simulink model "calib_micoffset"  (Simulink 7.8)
settings: Solver=FixedStepDiscrete  SolverMode=SingleTasking  StartTime=0.0  StopTime=inf  FixedStep=Ts  RelTol=1e-3
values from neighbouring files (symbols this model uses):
  amp_gain_factor = 0.73316    [hybrid_wind.m]    (also in measurements.m = 0.73312)
  Ampl_chirp = maxoutputvoltage/4    (= 1.25)    [measurements.m]
  Ampl_chirp_F = maxLSvolts*Bl/Re    [measurements.m]
  Ampl_chirp_U = maxoutputvoltage *amp_gain_factor*Bl/Re/(2*pi*fstop)*Sd/Mms    [measurements.m]
  HLL_d = c2d(HLL_c,Ts)    [hybrid_wind.m]    (also in measurements.m)
  maxoutputvoltage = 5    [hybrid_wind.m]    (also in measurements.m)
  sweep_time = runtime    (= 20)    [measurements.m]
  Ts = 25e-6    (= 2.5e-05)    [hybrid_wind.m]    (also in measurements.m)
undefined symbols (not defined in the file or in its folder): Bl, cell2mat, Mms, Re, Sd
libraries: dspsrcs4 x2, simulink x1

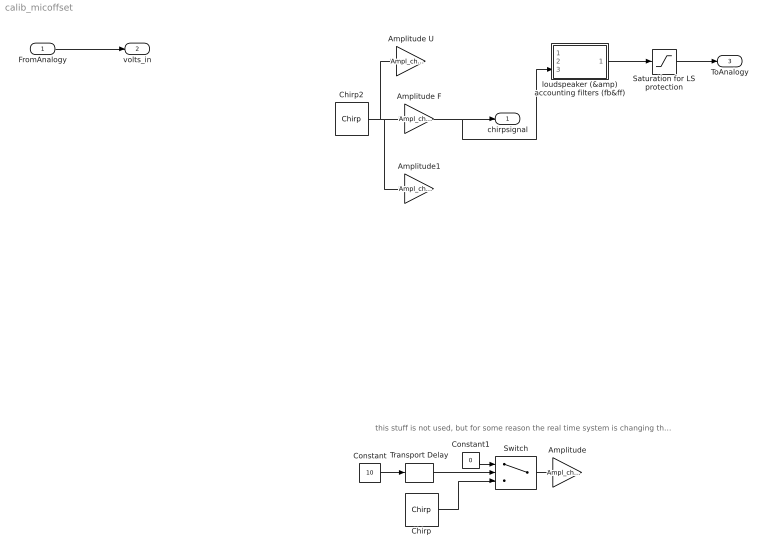
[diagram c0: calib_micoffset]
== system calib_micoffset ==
  note: this stuff is not used, but for some reason the real time system is changing the execution timing when the simulink patch is not complex enough!!
  FromAnalogy : Inport
  Amplitude : Gain  Gain=Ampl_chirp
  Amplitude F : Gain  Gain=Ampl_chirp_F
  Amplitude U : Gain  Gain=Ampl_chirp_U
  Amplitude1 : Gain  Gain=Ampl_chirp
  Chirp : dspsrcs4/Chirp  sweep=Linear  mode=Unidirectional  f0=fstart  f1=fstop  t1=sweep_time  Tsweep=sweep_time  phase=pi/2  Ts=Ts  spf=1  datatype=Single
  Chirp2 : dspsrcs4/Chirp  sweep=Linear  mode=Unidirectional  f0=fstart  f1=fstop  t1=sweep_time  Tsweep=sweep_time  phase=pi/2  Ts=Ts  spf=1  datatype=Double
  Constant : Constant  Value=10
  Constant1 : Constant  Value=0
  Saturation for LS protection : Saturate  UpperLimit=maxoutputvoltage  LowerLimit=-maxoutputvoltage
  Switch : Switch  Threshold=1
  Transport Delay : TransportDelay  DelayTime=sweep_time  BufferSize=8
  loudspeaker (&amp) accounting filters (fb&ff) : Subsystem
  chirpsignal : Outport
  volts_in : Outport  Port=2
  ToAnalogy : Outport  Port=3
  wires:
  FromAnalogy/1 -> volts_in/1
  Constant/1 -> Transport Delay/1
  Transport Delay/1 -> Switch/2
  Constant1/1 -> Switch/1
  Switch/1 -> Amplitude/1
  Chirp/1 -> Switch/3
  Amplitude/1 -> ?
  Chirp2/1 -> Amplitude F/1, Amplitude1/1, Amplitude U/1
  Saturation for LS protection/1 -> ToAnalogy/1
  loudspeaker (&amp) accounting filters (fb&ff)/1(V_amp_in) -> Saturation for LS protection/1
  Amplitude F/1 -> loudspeaker (&amp) accounting filters (fb&ff)/3(FLS), chirpsignal/1

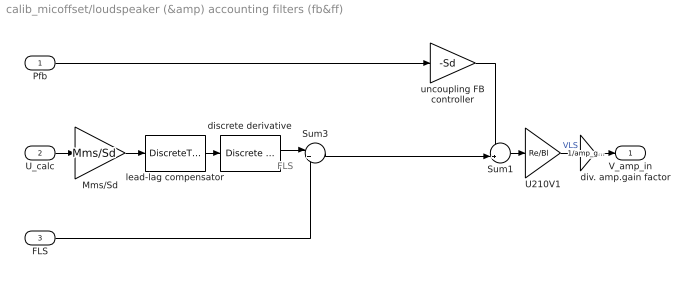
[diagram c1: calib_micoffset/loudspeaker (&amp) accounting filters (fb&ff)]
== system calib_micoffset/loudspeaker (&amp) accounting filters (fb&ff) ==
  note: FLS
  Pfb : Inport
  U_calc : Inport  Port=2
  FLS : Inport  Port=3
  Mms/Sd : Gain  Gain=Mms/Sd
  Sum1 : Sum  Inputs=-+|
  Sum3 : Sum  Inputs=|++
  U210V1 : Gain  Gain=Re/Bl
  discrete derivative : simulink/Discrete/Discrete Derivative  gainval=1.0  ICPrevScaledInput=0.0  InputProcessing=Inherited  OutMin=[]  OutMax=[]  OutDataType=fixdt(1, 16)  OutScaling=2^-10  DoSatur=off
  div. amp.gain factor : Gain  Gain=1/amp_gain_factor
  lead-lag compensator : DiscreteTransferFcn  Numerator=cell2mat(HLL_d.num)  Denominator=cell2mat(HLL_d.den)  SampleTime=Ts
  uncoupling FB controller : Gain  Gain=-Sd
  V_amp_in : Outport
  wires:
  Sum1/1 -> U210V1/1
  U210V1/1 -> div. amp.gain factor/1  "VLS"
  U_calc/1 -> Mms/Sd/1
  Pfb/1 -> uncoupling FB controller/1
  Mms/Sd/1 -> lead-lag compensator/1
  lead-lag compensator/1 -> discrete derivative/1
  div. amp.gain factor/1 -> V_amp_in/1
  Sum3/1 -> Sum1/2
  FLS/1 -> Sum3/2
  discrete derivative/1 -> Sum3/1
  uncoupling FB controller/1 -> Sum1/1
